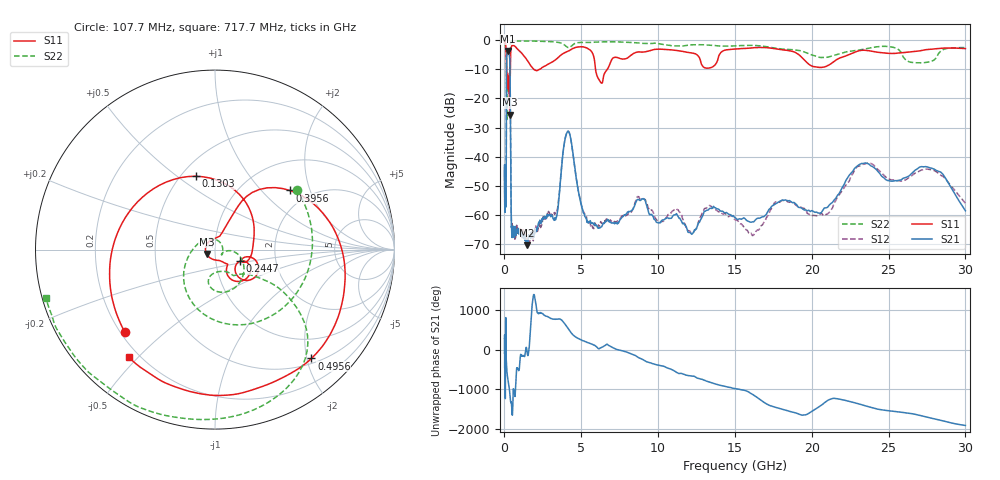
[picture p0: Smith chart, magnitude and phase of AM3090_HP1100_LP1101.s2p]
! Date/Time: Thu, Feb 28, 2019 2:07 PM
! Network Analyzer: Agilent Technologies E8364B Rev: A.07.50.67
! Sweep from 0.010 to 30.000 GHz, 1601 Points, Sweep Type: LOG
! Power Supply: 5.023 V, 0.002 A
# Hz S DB R 50
!freq MagS11 AngS11 MagS21 AngS21 MagS12 AngS12 MagS22 AngS22
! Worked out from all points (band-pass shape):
!   1601 points, 10 MHz to 30 GHz, reference 50 ohm
!   highest |S21| = -3.77 dB at 238.7 MHz (marker M1); lowest = -70.4 dB at 1.475 GHz (marker M2)
!   |S21| within 3 dB of the highest: 144.3 MHz to 348 MHz (203.7 MHz wide, 82.7 % of centre)
!   lowest |S11| = -25.5 dB at 342.2 MHz (marker M3), VSWR 1.11, Z = 45.4 - j2.17 ohm
!   |S11| at or under -10 dB: 136 MHz to 382.4 MHz (246.4 MHz wide, 95 % of centre); 1.899 GHz to 2.275 GHz (376.8 MHz wide, 18.1 % of centre); 5.925 GHz to 6.698 GHz (772.7 MHz wide, 12.2 % of centre)
!   |S22| runs from -27.2 to -0.1 dB; largest |S21 - S12| = 0.011
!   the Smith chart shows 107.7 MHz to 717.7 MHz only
!   S11 on the Smith chart (normalised r, x): 107.7 MHz: 0.22, -0.37; 130.3 MHz: 0.59, +0.59; 244.7 MHz: 1.31, -0.17; 395.6 MHz: 1.60, +1.47; 495.6 MHz: 0.59, -2.09; 717.7 MHz: 0.16, -0.47
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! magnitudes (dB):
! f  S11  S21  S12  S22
! 10 MHz  -0.3  -47.9  -45.2  -0.7
! 38.04 MHz  -0.4  -57.4  -57.0  -1.5
! 107.7 MHz  -3.4  -55.5  -52.2  -5.0
! 130.3 MHz  -7.5  -17.9  -17.8  -8.7
! 144.7 MHz  -13.2  -6.7  -6.6  -26.6
! 238.7 MHz  -16.8  -3.8  -3.7  -16.0
! 244.7 MHz  -16.3  -3.8  -3.7  -16.8
! 342.2 MHz  -25.5  -6.2  -6.2  -12.2
! 395.6 MHz  -5.5  -31.7  -31.4  -1.5
! 443.9 MHz  -2.4  -61.6  -60.5  -0.4
! 495.6 MHz  -1.8  -66.0  -63.1  -0.2
! 550.5 MHz  -1.8  -64.8  -66.6  -0.2
! 717.7 MHz  -2.3  -66.8  -66.5  -0.2
! 1.475 GHz  -6.9  -70.4  -68.5  -0.3
! 2.084 GHz  -10.5  -65.7  -64.4  -0.4
! 3.352 GHz  -6.6  -61.3  -58.9  -0.7
! 4.115 GHz  -3.9  -31.4  -31.3  -2.5
! 5.338 GHz  -2.7  -61.3  -60.6  -0.8
! 7.926 GHz  -6.3  -59.7  -60.2  -0.7
! 16.21 GHz  -2.6  -62.4  -67.0  -1.8
! 23.48 GHz  -3.5  -42.2  -42.4  -3.0
! 30 GHz  -2.9  -58.6  -56.0  -2.6
